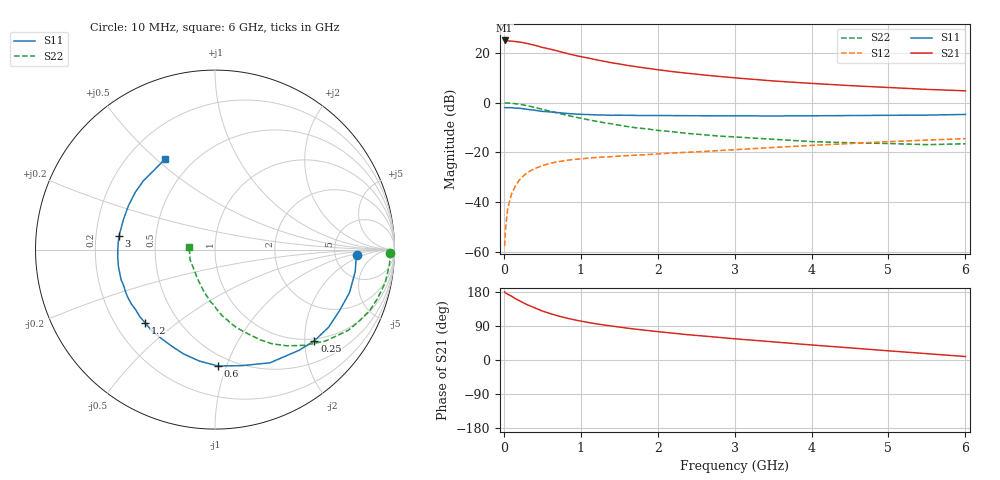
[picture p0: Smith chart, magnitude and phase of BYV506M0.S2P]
! SIEMENS Small Signal Semiconductors
! BFY420
! Si NPN RF SIEGET Grounded Emitter Transistor in MICRO-X
! VCE = 0.5 V  IC = 6 mA
! Common Emitter S-Parameters:  October  1996
# GHz  S  MA  R  50
!  f  S11  S21  S12  S22
! GHz  MAG  ANG  MAG  ANG  MAG  ANG  MAG  ANG
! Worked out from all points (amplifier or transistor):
!   36 points, 10 MHz to 6 GHz, reference 50 ohm
!   highest |S21| = 24.9 dB at 10 MHz (marker M1)
!   |S21| within 3 dB of that: start of sweep to 531.6 MHz
!   unconditionally stable (mu >= 1): 2.734 GHz to end of sweep
!   at 250 MHz: K = 0.13, MSG = 26.8 dB, |S12| = -29.6 dB
!   at 1.4 GHz: K = 0.63, MSG = 18.9 dB, |S12| = -21.8 dB
!   at 6 GHz: K = 1.17, MAG = 7.1 dB, |S12| = -14.5 dB
!   S11 on the Smith chart (normalised r, x): 10 MHz: 8.39, -1.30; 250 MHz: 0.95, -2.22; 600 MHz: 0.42, -0.94; 1.2 GHz: 0.33, -0.39; 3 GHz: 0.30, +0.07; 6 GHz: 0.35, +0.53
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0.01  0.7915 -2.1  17.65 179.8  0.0013 103.1  0.9774 -1.0
0.02  0.7879 -3.8  17.64 177.3  0.0027 81.3  0.9791 -2.1
0.05  0.7908 -8.9  17.26 173.6  0.0074 83.7  0.9744 -5.5
0.1  0.7869 -17.7  17.12 168.5  0.0145 81.2  0.9663 -11.0
0.15  0.7728 -25.9  16.76 161.8  0.0211 75.3  0.9462 -16.6
0.25  0.7513 -42.5  15.96 151.2  0.033 68.2  0.8953 -26.6
0.3  0.7309 -50.1  15.37 146.2  0.0386 65.2  0.8675 -31.3
0.4  0.7013 -64.1  14.15 137.8  0.047 58.3  0.799 -39.6
0.5  0.6637 -76.9  12.82 129.2  0.054 52.7  0.7324 -46.7
0.6  0.6488 -88.4  11.83 122.7  0.0601 48.8  0.6706 -53.1
0.7  0.6273 -97.9  10.83 116.6  0.0645 45.2  0.6154 -58.6
0.8  0.607 -106.8  9.85 111.4  0.068 42.1  0.5634 -63.3
0.9  0.5893 -114.3  9.023 106.7  0.0716 39.8  0.5204 -67.0
1.1  0.573 -128.2  7.801 98.9  0.0763 37.0  0.4502 -74.6
1.2  0.5639 -133.7  7.231 95.5  0.0786 35.9  0.4204 -77.9
1.6  0.554 -151.6  5.582 84.1  0.0857 32.8  0.3309 -88.6
2.2  0.5462 -170.1  4.16 70.8  0.0968 31.0  0.2582 -101.1
3  0.5401 171.8  3.133 56.0  0.1127 29.2  0.2036 -115.3
3.5  0.5369 161.7  2.712 47.9  0.1249 27.6  0.1827 -124.1
4.5  0.5471 144.2  2.186 32.0  0.1502 22.1  0.1553 -143.1
5.5  0.5584 126.9  1.836 16.7  0.1761 15.0  0.1424 -171.9
6  0.5763 119.0  1.718 9.2  0.1881 11.0  0.1483 173.4
